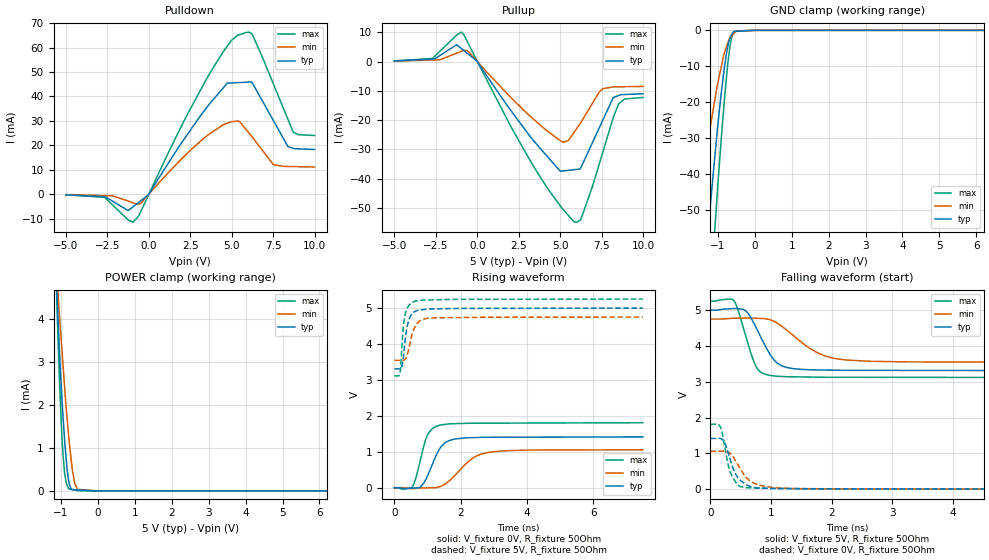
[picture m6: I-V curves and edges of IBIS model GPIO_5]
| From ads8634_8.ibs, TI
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|   GPIO_5   5V digital input Model
[Model] GPIO_5   | 5V digital input
Model_type   I/O
Polarity   Non-Inverting
Vinl = 1.5
Vinh = 3.5
Vmeas = 2.5
Vref = 2.5
Cref = 15pF
Rref = 50
|   typ   min   max
|   (nom PVT)   (Fast PVT)   (slow PVT)
|BUFFER as INPUT
|C_comp from L-C Tank method(L=1nH)
|Resonant Frequency(Hz)   4.03G   4.24G   3.52G
|C_comp   1.5563E-12   1.4128E-12   2.05155E-12
|BUFFER OUTPUT TURNED HIGH
|C_comp from L-C Tank method(L=1nH)
|Resonant Frequency(Hz)   4.39G   4.39G   3.67G
|C_comp   1.3185E-12   1.3185E-12   1.88842E-12
|BUFFER OUTPUT TURNED LOW
|C_comp from L-C Tank method(L=1nH)
|Resonant Frequency(Hz)   4.43G   4.47G   3.73G
C_comp   1.29444E-12   1.26992E-12   1.82004E-12
| Where   nom PVT is  Nominal Process, 5V, 25C
|   Fast PVT is Strong Process, 4.5V, -40C
|   Slow PVT is Weak Process, 5.5V, 85C
|C_comp - from L-C Tank method, L = 1nH, peak frequency
[Model Spec]   | 5V
Vinl   1.5   1.35   1.65
Vinh   3.5   3.15   3.85
|Vinl = 0.3 DVDD
|Vinh = 0.7 DVDD
[Voltage Range]   5   4.75   5.25
[Temperature Range]   27   125   -40
[Pullup Reference]   5   4.75   5.25
[Pulldown Reference]   0   0   0
[Power Clamp Reference]   5   4.75   5.25
[GND Clamp Reference]   0   0   0
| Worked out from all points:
|   slope of the pulldown table from 0 to 0.75 V, typ, clamps not added: 91.5 ohm
|   slope of the pullup table from 0 to 0.75 V, typ, clamps not added: 118 ohm
|   GND clamp passes 1 mA (typ) near -0.62 V on its own axis
|   POWER clamp passes 1 mA (typ) near -0.88 V on its own axis
|   falling waveform, V_fixture 5V, R_fixture 50Ohm: 20-80 % time 325ps typ, 588ps min, 234ps max; typ from 5 V to 3.31 V
|   rising waveform, V_fixture 0V, R_fixture 50Ohm: 20-80 % time 425ps typ, 721ps min, 313ps max; typ from 0.002 V to 1.42 V
|   rising waveform, V_fixture 5V, R_fixture 50Ohm: 20-80 % time 163ps typ, 226ps min, 124ps max; typ from 3.31 V to 5 V
|   falling waveform, V_fixture 0V, R_fixture 50Ohm: 20-80 % time 199ps typ, 278ps min, 151ps max; typ from 1.42 V to 0.003 V
[Pulldown]
|   Voltage   I(typ)   I(min)   I(max)
-5V       -226.1uA   -151.2uA   -226.9uA
-2.671V   -1.023mA   -542.3uA   -1.236mA
-953.8mV  -5.125mA   -3.531mA   -11.43mA
-13.55mV  -145.4uA   -104.2uA   -190.7uA
3.637V    36.78mA    24.56mA    49.02mA
4.727V    45.43mA    29.05mA    60.57mA
5.39V     45.66mA    30mA       65.06mA
5.858V    45.82mA    26.52mA    66.15mA
6.263V    45.24mA    23.15mA    65.04mA
7.511V    30.12mA    12.06mA    45.08mA
8.707V    18.79mA    11.31mA    25.44mA
9.985V    18.32mA    11.16mA    24.03mA
[GND Clamp]
|   Voltage   I(typ)   I(min)   I(max)
-5V       -576.4mA   -401.2mA   -708.5mA
-1.67V    -106.8mA   -61.97mA   -151.3mA
-1.518V   -87.19mA   -49.42mA   -126.2mA
-1.248V   -53.71mA   -29.76mA   -81.64mA
-1.101V   -37.41mA   -20.59mA   -58.34mA
-1.023V   -28.81mA   -15.8mA    -46.72mA
-814.1mV  -9.77mA    -6.015mA   -18.54mA
-727.9mV  -4.504mA   -3.507mA   -9.135mA
-672.4mV  -2.247mA   -2.123mA   -4.548mA
-571.4mV  -324.9uA   -977.7uA   -723.3uA
-30.07mV  -14.74uA   -2.884uA   -15.06uA
9.985V    0A         0A         0A
[Pullup]
|   Voltage   I(typ)   I(min)   I(max)
-5V       186.9uA    141uA      205.2uA
-2.703V   833uA      520.5uA    1.055mA
-1.248V   5.752mA    2.837mA    9.018mA
-829.2mV  3.84mA     3.809mA    9.366mA
2.062V    -17.01mA   -12.48mA   -22.59mA
4.973V    -37.25mA   -26.86mA   -49.06mA
5.858V    -36.91mA   -23.99mA   -54.75mA
6.27V     -35.92mA   -20.59mA   -53.52mA
7.533V    -20.45mA   -9.336mA   -31.61mA
8.193V    -12.37mA   -8.65mA    -19.22mA
8.533V    -11.56mA   -8.622mA   -14.38mA
9.985V    -10.99mA   -8.504mA   -12.26mA
[POWER Clamp]
|   Voltage   I(typ)   I(min)   I(max)
-5V       100.8mA    79.3mA     128.3mA
-1.237V   7.385mA    7.149mA    7.989mA
-1.089V   4.197mA    4.825mA    3.82mA
-1.077V   3.949mA    4.634mA    3.507mA
-987.9mV  2.399mA    3.471mA    1.534mA
-941.7mV  1.709mA    2.923mA    832.5uA
-898.2mV  1.165mA    2.405mA    407uA
-834mV    513.6uA    1.709mA    139.4uA
-793.8mV  262uA      1.325mA    50.57uA
-685.5mV  31.21uA    466.7uA    31.67uA
-556.8mV  25.23uA    36.99uA    9.191uA
9.985V    0A         0A         0A
[Ramp]
R_load = 50
|   typ   min   max
dV/dt_r   0.847963/4.24303e-010  0.632809/7.18809e-010   1.08519/3.12765e-010
dV/dt_f   1.01404/3.23476e-010  0.721415/5.8388e-010   1.28164/2.33948e-010
[Falling Waveform]
V_fixture = 5V
V_fixture_min = 4.75V
V_fixture_max = 5.25V
R_fixture = 50Ohm
C_fixture = 0F
|   Time   V(typ)   V(min)   V(max)
0s        4.999V     4.749V     5.25V
388.1ps   5.043V     4.773V     5.266V
569.8ps   4.998V     4.78V      4.357V
746.3ps   4.54V      4.773V     3.455V
830.8ps   4.251V     4.767V     3.266V
979.9ps   3.781V     4.736V     3.177V
1.25ns    3.402V     4.455V     3.141V
1.766ns   3.33V      3.81V      3.129V
2.242ns   3.319V     3.608V     3.125V
7.5ns     3.309V     3.546V     3.114V
[Rising Waveform]
V_fixture = 0V
V_fixture_min = 0V
V_fixture_max = 0V
R_fixture = 50Ohm
C_fixture = 0F
|   Time   V(typ)   V(min)   V(max)
0s        2.5mV      2.517mV    894.5uV
538.9ps   -8.685mV   -25.68mV   22.65mV
655.9ps   -6.641mV   -17.72mV   297.6mV
793.7ps   29.85mV    -7.045mV   806.5mV
985.7ps   305.9mV    -3.452mV   1.443V
1.368ns   1.089V     26.28mV    1.743V
1.804ns   1.352V     324.2mV    1.783V
2.369ns   1.395V     828.1mV    1.796V
2.877ns   1.405V     989.3mV    1.797V
7.5ns     1.416V     1.057V     1.81V
[Rising Waveform]
V_fixture = 5V
V_fixture_min = 4.75V
V_fixture_max = 5.25V
R_fixture = 50Ohm
C_fixture = 0F
|   Time   V(typ)   V(min)   V(max)
0s        3.309V     3.546V     3.114V
167.6ps   3.308V     3.545V     3.183V
223.1ps   3.363V     3.545V     3.874V
264.3ps   3.578V     3.547V     4.413V
337.9ps   4.206V     3.59V      4.872V
447.2ps   4.694V     3.921V     5.086V
630.9ps   4.91V      4.495V     5.195V
854.1ps   4.954V     4.683V     5.219V
1.184ns   4.977V     4.728V     5.228V
7.5ns     4.999V     4.748V     5.25V
[Falling Waveform]
|Gnd
V_fixture = 0V
V_fixture_min = 0V
V_fixture_max = 0V
R_fixture = 50Ohm
C_fixture = 0F
|   Time   V(typ)   V(min)   V(max)
0s        1.416V     1.058V     1.81V
161.3ps   1.419V     1.059V     1.753V
234.9ps   1.3V       1.059V     1.206V
286.8ps   1.054V     1.04V      728.9mV
332.2ps   798.1mV    989.3mV    459.4mV
443.4ps   344.6mV    710.2mV    136.2mV
556.8ps   171.1mV    403.4mV    49.53mV
811.9ps   35.02mV    111.9mV    27.63mV
1.394ns   15.05mV    16.62mV    17.71mV
7.5ns     2.536mV    2.822mV    895.6uV
